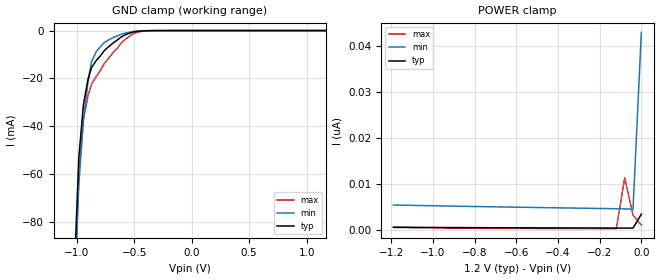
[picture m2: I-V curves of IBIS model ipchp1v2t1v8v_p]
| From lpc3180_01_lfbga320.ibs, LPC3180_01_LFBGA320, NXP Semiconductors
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| |   Rev 0.20 IBIS Model Design Automation Generation   |
| |   N O N - S I L I C O N   C O R R E L A T E D   |
| |   This IBIS [Model] is pre-Beta tactical support   |
| |  Note: this IBIS [Model] contains clamp curves generated   |
| |   through simulation which should not be relied upon   |
| ipchp1v2t1v8v
|   Input Pad 1v2
|   Push Pull
|   CMOS
|   Programmable between
|   - (p1=0, p2=1) plain input
|   - (p1=0, p2=0) with Pull Up
|   - (p1=1, p2=1) with Pull Down
|   - (p1=1, p2=0) with Repeater
|   Characterized at Core 1.2V and I/O 1.8V
| Plain input Mode (p1=0, p2=1)
[Model]   ipchp1v2t1v8v_p | of ipchp1v2t1v8v
Model_type   Input
|  Reciever Thresholds
Vinl   = 0.36V
Vinh   = 0.84V
| [Process Range]   typical   min   max
| C_comp edge width   400.000ps   400.000ps   400.000ps
| C_comp Tstrobe   40.000fs   40.000fs   40.000fs
C_comp   2.020pF   1.889pF   2.187pF
[Temperature Range]   25   105   -20
[Voltage Range]   1.20V   1.10V   1.30V
[GND Clamp Reference]   0.00V   0.00V   0.00V
[Pulldown Reference]   0.00V   0.00V   0.00V
[POWER Clamp Reference]   1.20V   1.10V   1.30V
[Pullup Reference]   1.20V   1.10V   1.30V
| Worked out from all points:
|   GND clamp passes 1 mA (typ) near -0.53 V on its own axis
[GND Clamp]
| ref voltage   0.00V   0.00V   0.00V
|   Voltage   I(typ)   I(min)   I(max)
-1.2V     -373.8mA   -377.3mA   -396.4mA
-1.01V    -89.18mA   -101.8mA   -99.48mA
-980mV    -53.06mA   -64.22mA   -60.46mA
-940mV    -30.85mA   -37.28mA   -37.22mA
-900mV    -20.29mA   -21.21mA   -27.1mA
-870mV    -15.46mA   -12.99mA   -22.45mA
-830mV    -12.6mA    -8.908mA   -19.25mA
-760mV    -8.421mA   -5.036mA   -13.86mA
-570mV    -1.644mA   -980.1uA   -3.422mA
-500mV    -495.7uA   -383.2uA   -1.141mA
-420mV    -119.8uA   -130uA     -229.2uA
1.17V     1.269nA    4.483nA    153.6pA
[Power Clamp]   | Vtable = Vcc - Vpad
| ref voltage   1.20V   1.10V   1.30V
|   Voltage   I(typ)   I(min)   I(max)
-1.19V    514.6pA    5.355nA    470.7pA
-120mV    324.1pA    4.532nA    199.8pA
-80mV     319.7pA    4.497nA    11.28nA
-40mV     314.7pA    4.436nA    3.166nA
0V        3.36nA     42.94nA    983.3pA
